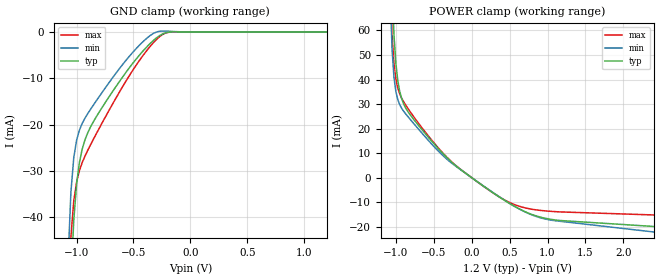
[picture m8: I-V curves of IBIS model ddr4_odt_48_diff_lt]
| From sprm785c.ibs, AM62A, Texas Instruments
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|   Model ddr4_odt_48_diff_lt
[Model] ddr4_odt_48_diff_lt
Model_type Input
Polarity   Non-Inverting
Enable   Active-High
Vinl =  0.700V
Vinh =  0.900V
C_comp   2.297pF   2.106pF   2.453pF
[Model Spec]
Vinh   0.900V   0.820V   0.980V
Vinl   0.700V   0.620V   0.780V
[Temperature Range]   25.000   -40.000   -40.000
[Voltage Range]   1.200V   1.140V   1.260V
[C Comp Corner]
C_comp   2.297pF   2.106pF   2.453pF
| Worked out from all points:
|   GND clamp passes 1 mA (typ) near -0.28 V on its own axis
|   POWER clamp passes 1 mA (typ) near -0.04 V on its own axis
[GND_clamp]
|Voltage   I(typ)   I(min)   I(max)
-1.2V     -386.1mA   -350.8mA   -362.7mA
-1.075V   -76.68mA   -49.36mA   -59.37mA
-1.05V    -54.32mA   -34.63mA   -44.31mA
-1.025V   -40.8mA    -27.21mA   -36.55mA
-1V       -32.88mA   -23.38mA   -32.41mA
-975mV    -28.18mA   -21.18mA   -29.91mA
-950mV    -25.22mA   -19.71mA   -28.15mA
-875mV    -20.39mA   -16.61mA   -24.24mA
-750mV    -15.33mA   -12.16mA   -18.49mA
-350mV    -2.413mA   -719uA     -3.022mA
-175mV    -1.651uA   133.6uA    -19.26uA
1.2V      0A         0A         0A
[POWER_clamp]
|Voltage   I(typ)   I(min)   I(max)
-1.2V     599mA      617.4mA    626.4mA
-1.075V   110.9mA    74.8mA     81.19mA
-1.05V    78.04mA    52.21mA    58.11mA
-1.025V   58.25mA    40.91mA    46.37mA
-1V       46.6mA     35.11mA    40.15mA
-975mV    39.64mA    31.86mA    36.54mA
-900mV    30.28mA    27.19mA    31.06mA
-350mV    8.895mA    8.167mA    9.06mA
250mV     -5.483mA   -5.407mA   -5.558mA
575mV     -11.87mA   -11.85mA   -11.09mA
950mV     -16.41mA   -16.7mA    -13.48mA
2.4V      -19.89mA   -22.13mA   -15.19mA
